// Version 2.0, 05.09.99: Änderungen:
// Umstrukturierungen und Bearbeitungzeitoptimierung,
// Quittierung von DB71-Aufträgen sofort
// FC90_4

FUNCTION FC 90 : VOID
TITLE = ANSTEUERUNG QUIT_WZV
VERSION : 2.0

BEGIN
NETWORK
TITLE =Quittung Werkzeug beladen beendet Magazin
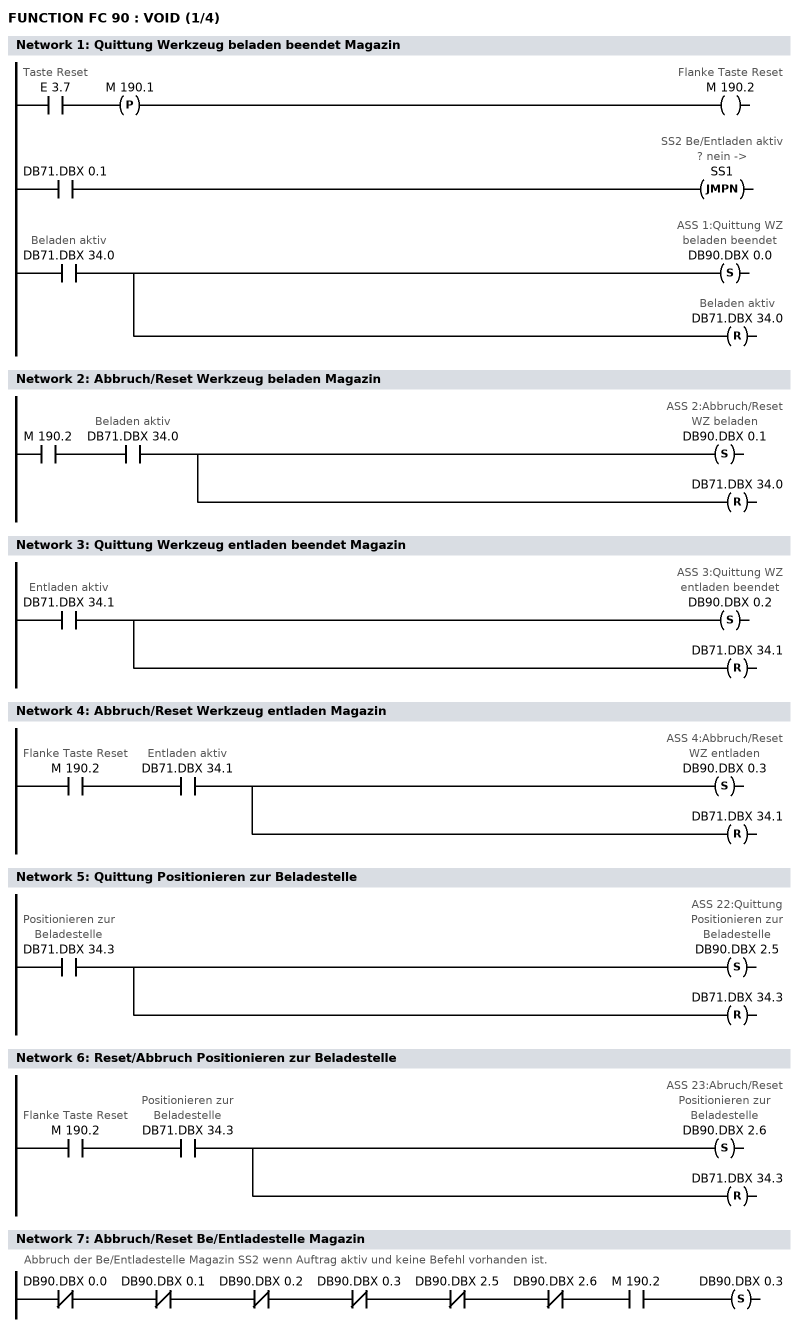
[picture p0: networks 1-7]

      U     E      3.7; // Taste Reset
      FP    M    190.1;
      =     M    190.2; // Flanke Taste Reset
	U	DB71.DBX	0.1;
	SPBN  SS1; // SS2 Be/Entladen aktiv ? nein ->
      U     DB71.DBX   34.0; // Beladen aktiv
//    U     M    190.0; // Flanke beladen Magazin beendet
      S     DB90.DBX    0.0; // ASS 1:Quittung WZ beladen beendet
	R	DB71.DBX   34.0; // Beladen aktiv
NETWORK
TITLE =Abbruch/Reset Werkzeug beladen Magazin

      U     M    190.2;
      U     DB71.DBX   34.0; // Beladen aktiv
      S     DB90.DBX    0.1; // ASS 2:Abbruch/Reset WZ beladen
	R	DB71.DBX   34.0;
NETWORK
TITLE =Quittung Werkzeug entladen beendet Magazin

      U     DB71.DBX   34.1; // Entladen aktiv
//    U     M    190.3; // Flanke entladen Magazin beendet
      S     DB90.DBX    0.2; // ASS 3:Quittung WZ entladen beendet
	R	DB71.DBX	34.1;
NETWORK
TITLE =Abbruch/Reset Werkzeug entladen Magazin

      U     M    190.2; // Flanke Taste Reset
      U     DB71.DBX   34.1; // Entladen aktiv
      S     DB90.DBX    0.3; // ASS 4:Abbruch/Reset WZ entladen
	R	DB71.DBX   34.1;

NETWORK
TITLE =Quittung Positionieren zur Beladestelle

      U     DB71.DBX   34.3;  // Positionieren zur Beladestelle
//    U     M    193.2; // Positionieren beendet
      S     DB90.DBX    2.5; // ASS 22:Quittung Positionieren zur Beladestelle
	R	DB71.DBX   34.3;
NETWORK
TITLE =Reset/Abbruch Positionieren zur Beladestelle

      U     M    190.2; // Flanke Taste Reset
      U     DB71.DBX   34.3; // Positionieren zur Beladestelle
      S     DB90.DBX    2.6; // ASS 23:Abruch/Reset Positionieren zur Beladestelle
	R	DB71.DBX   34.3;
NETWORK
TITLE =Abbruch/Reset Be/Entladestelle Magazin
//Abbruch der Be/Entladestelle Magazin SS2 wenn Auftrag aktiv und keine Befehl vorhanden ist.

      UN    DB90.DBX    0.0;
      UN    DB90.DBX    0.1;
      UN    DB90.DBX    0.2;
	UN	DB90.DBX	0.3;
	UN    DB90.DBX    2.5;
      UN	DB90.DBX	2.6;
      U     M 	190.2;
      S     DB90.DBX    0.3;
NETWORK
TITLE =Quittung Werkzeug beladen beendet Spindel
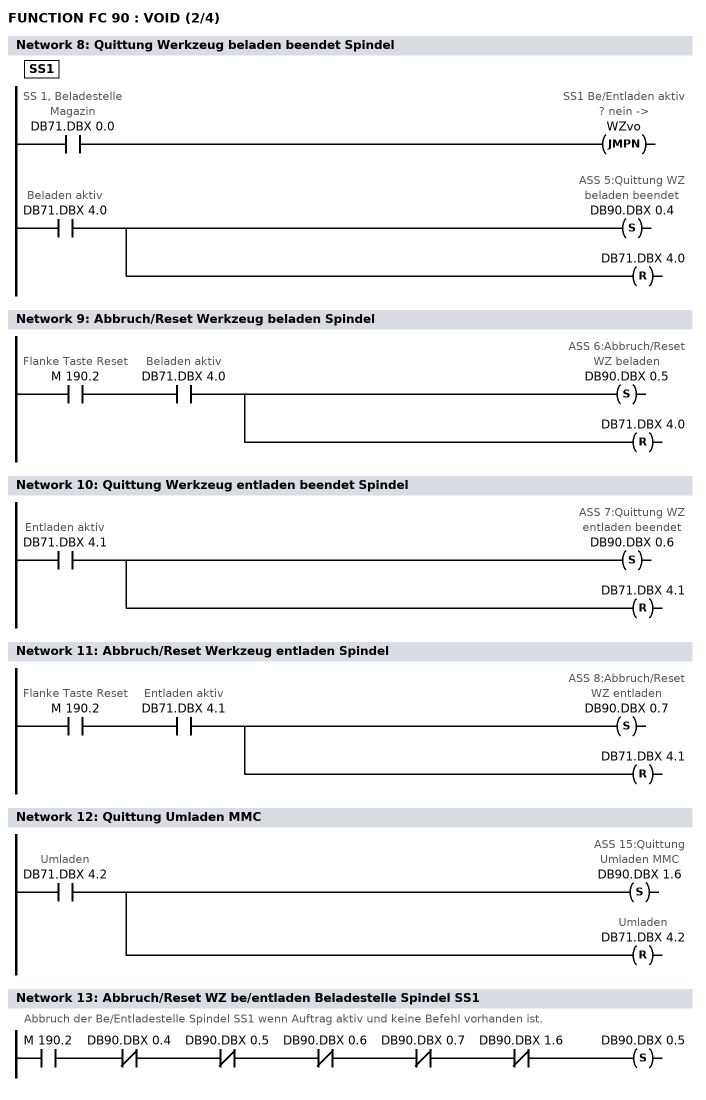
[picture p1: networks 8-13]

SS1:  U     DB71.DBX    0.0; // SS 1, Beladestelle Magazin
	SPBN  WZvo; // SS1 Be/Entladen aktiv ? nein ->
      U     DB71.DBX    4.0; // Beladen aktiv
//    U     M    193.0; // Flanke beladen Spindel beendet
      S     DB90.DBX    0.4; // ASS 5:Quittung WZ beladen beendet
	R	DB71.DBX	4.0;
NETWORK
TITLE =Abbruch/Reset Werkzeug beladen Spindel

      U     M    190.2; // Flanke Taste Reset
      U     DB71.DBX    4.0; // Beladen aktiv
      S     DB90.DBX    0.5; // ASS 6:Abbruch/Reset WZ beladen
      R     DB71.DBX    4.0;
NETWORK
TITLE =Quittung Werkzeug entladen beendet Spindel

      U     DB71.DBX    4.1; // Entladen aktiv
//    U     M    193.1; // Flanke entladen beendet
      S     DB90.DBX    0.6; // ASS 7:Quittung WZ entladen beendet
	R     DB71.DBX    4.1;
NETWORK
TITLE =Abbruch/Reset Werkzeug entladen Spindel

      U     M    190.2; // Flanke Taste Reset
      U     DB71.DBX    4.1; // Entladen aktiv
      S     DB90.DBX    0.7; // ASS 8:Abbruch/Reset WZ entladen
      R     DB71.DBX    4.1;
NETWORK
TITLE =Quittung Umladen MMC

      U     DB71.DBX    4.2; // Umladen
      S     DB90.DBX    1.6; // ASS 15:Quittung Umladen MMC
	R     DB71.DBX    4.2; // Umladen

NETWORK
TITLE =Abbruch/Reset WZ be/entladen Beladestelle Spindel SS1
//Abbruch der Be/Entladestelle Spindel SS1 wenn Auftrag aktiv und keine Befehl vorhanden ist.

      U	M	190.2;
      UN    DB90.DBX    0.4;
      UN    DB90.DBX    0.5;
      UN    DB90.DBX    0.6;
 	UN    DB90.DBX    0.7;
      UN    DB90.DBX    1.6;
      S     DB90.DBX    0.5;

NETWORK
TITLE =Quittung Wechsel vorbereiten beendet
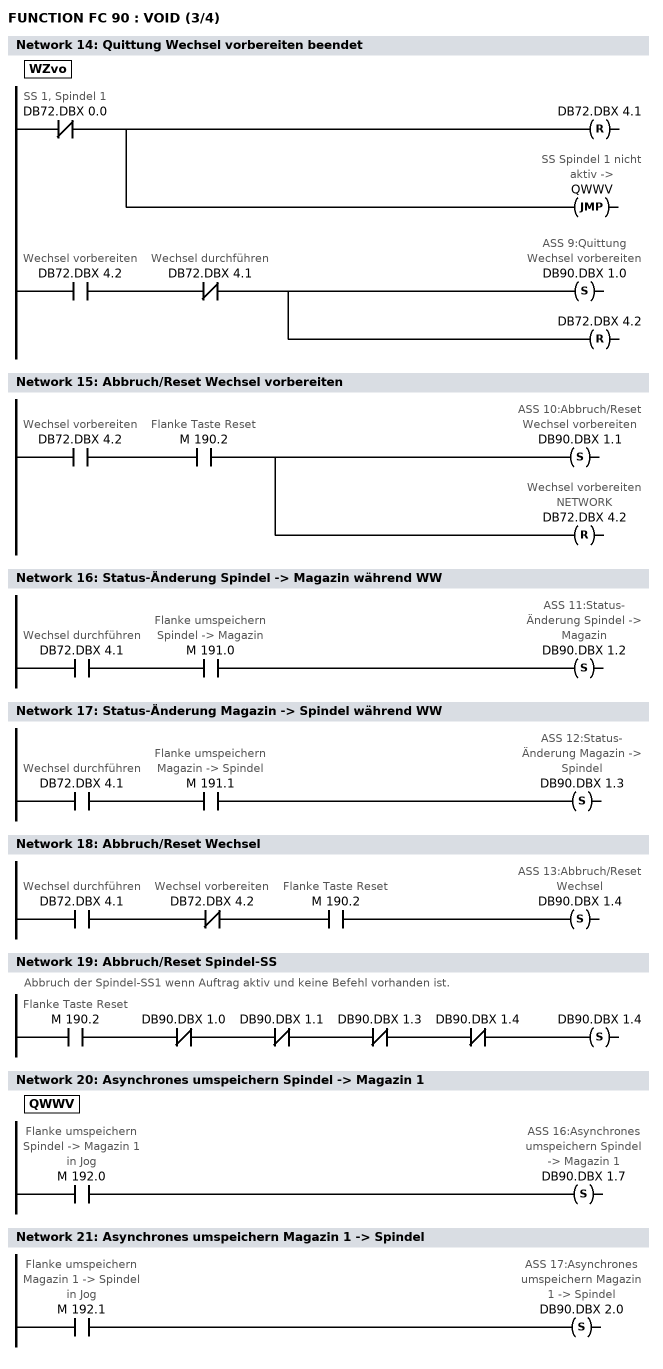
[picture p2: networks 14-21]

WZvo: UN	DB72.DBX	0.0; // SS 1, Spindel 1
	R	DB72.DBX	4.1;
      SPB  QWWV; // SS Spindel 1 nicht aktiv ->
	U     DB72.DBX    4.2; // Wechsel vorbereiten
      UN    DB72.DBX    4.1; // Wechsel durchführen
//    U     M    190.4; // Flanke Wechsel vorbereitet beendet
      S     DB90.DBX    1.0; // ASS 9:Quittung Wechsel vorbereiten
      R	DB72.DBX	4.2;
NETWORK
TITLE =Abbruch/Reset Wechsel vorbereiten

      U     DB72.DBX    4.2; // Wechsel vorbereiten
      U     M    190.2; // Flanke Taste Reset
      S     DB90.DBX    1.1; // ASS 10:Abbruch/Reset Wechsel vorbereiten
      R     DB72.DBX    4.2; // Wechsel vorbereitenNETWORK
NETWORK
TITLE =Status-Änderung Spindel -> Magazin während WW

      U     DB72.DBX    4.1; // Wechsel durchführen
      U     M    191.0; // Flanke umspeichern Spindel -> Magazin
      S     DB90.DBX    1.2; // ASS 11:Status-Änderung Spindel -> Magazin
NETWORK
TITLE =Status-Änderung Magazin -> Spindel während WW

      U     DB72.DBX    4.1; // Wechsel durchführen
      U     M    191.1; // Flanke umspeichern Magazin -> Spindel
      S     DB90.DBX    1.3; // ASS 12:Status-Änderung Magazin -> Spindel
NETWORK
TITLE =Abbruch/Reset Wechsel

      U     DB72.DBX    4.1; // Wechsel durchführen
      UN    DB72.DBX    4.2; // Wechsel vorbereiten
      U     M    190.2; // Flanke Taste Reset
      S     DB90.DBX    1.4; // ASS 13:Abbruch/Reset Wechsel
NETWORK
TITLE =Abbruch/Reset Spindel-SS
//Abbruch der Spindel-SS1 wenn Auftrag aktiv und keine Befehl vorhanden ist.

	U	M 	190.2; // Flanke Taste Reset
	UN	DB90.DBX	1.0;
      UN    DB90.DBX    1.1;
	UN	DB90.DBX	1.3;
      UN    DB90.DBX    1.4;
      S     DB90.DBX    1.4;
NETWORK
TITLE =Asynchrones umspeichern Spindel -> Magazin 1

QWWV: U     M    192.0; // Flanke umspeichern Spindel -> Magazin 1 in Jog
      S     DB90.DBX    1.7; // ASS 16:Asynchrones umspeichern Spindel -> Magazin 1
NETWORK
TITLE =Asynchrones umspeichern Magazin 1 -> Spindel

      U     M    192.1; // Flanke umspeichern Magazin 1 -> Spindel in Jog
      S     DB90.DBX    2.0; // ASS 17:Asynchrones umspeichern Magazin 1 -> Spindel
NETWORK
TITLE =Asynchrones umspeichern Spindel -> Magazin 2
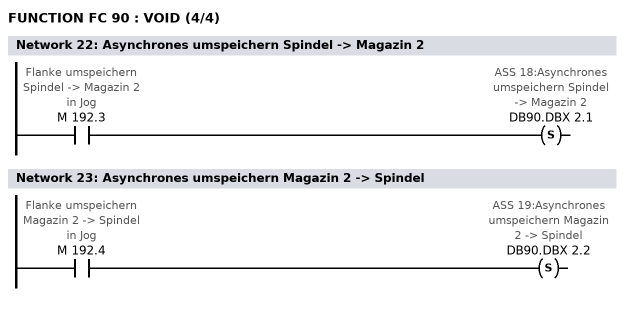
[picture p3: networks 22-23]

      U     M    192.3; // Flanke umspeichern Spindel -> Magazin 2 in Jog
      S     DB90.DBX    2.1; // ASS 18:Asynchrones umspeichern Spindel -> Magazin 2
NETWORK
TITLE =Asynchrones umspeichern Magazin 2 -> Spindel

      U     M    192.4; // Flanke umspeichern Magazin 2 -> Spindel in Jog
      S     DB90.DBX    2.2; // ASS 19:Asynchrones umspeichern Magazin 2 -> Spindel
NETWORK
TITLE =Änderung Istposition Magazin 1
// In MW180 steht die aktuelle Istposition der Wechselstelle MAG 1 in Format Int (ist
// vom Anwender zu versorgen).
	L     DB90.DBW   10; // Istposition alt
      L     MW   180; // Istposition neu
      T     DB90.DBW   10;
      <>I   ;
      S     DB90.DBX    2.3; // ASS 20: Änderung Istposition Magazin
NETWORK
TITLE =Änderung Istposition Magazin 2
// In MW184 steht die aktuelle Istposition der Wechselstelle MAG 2 in Format Int (ist
// vom Anwender zu versorgen).
	L     DB90.DBW   12; // Istposition MAG 2 alt
      L     MW   184; // Istposition MAG 2 neu
      T     DB90.DBW   12;
      <>I   ;
      S     DB90.DBX    2.4; // ASS 21: Änderung Istposition Magazin
NETWORK
TITLE =Fehlerbit löschen

      U     M    192.7; // Taste Fehler löschen
      R     DB90.DBX    4.0; // Fehler Quittung FC 8
NETWORK
TITLE =Aufruf FB 90
// Aufruf nur wenn QUIT_1 (FB90, DB90) bereits übersetzt wurde.
      CALL FB    90 , DB    90 ;

END_FUNCTION

